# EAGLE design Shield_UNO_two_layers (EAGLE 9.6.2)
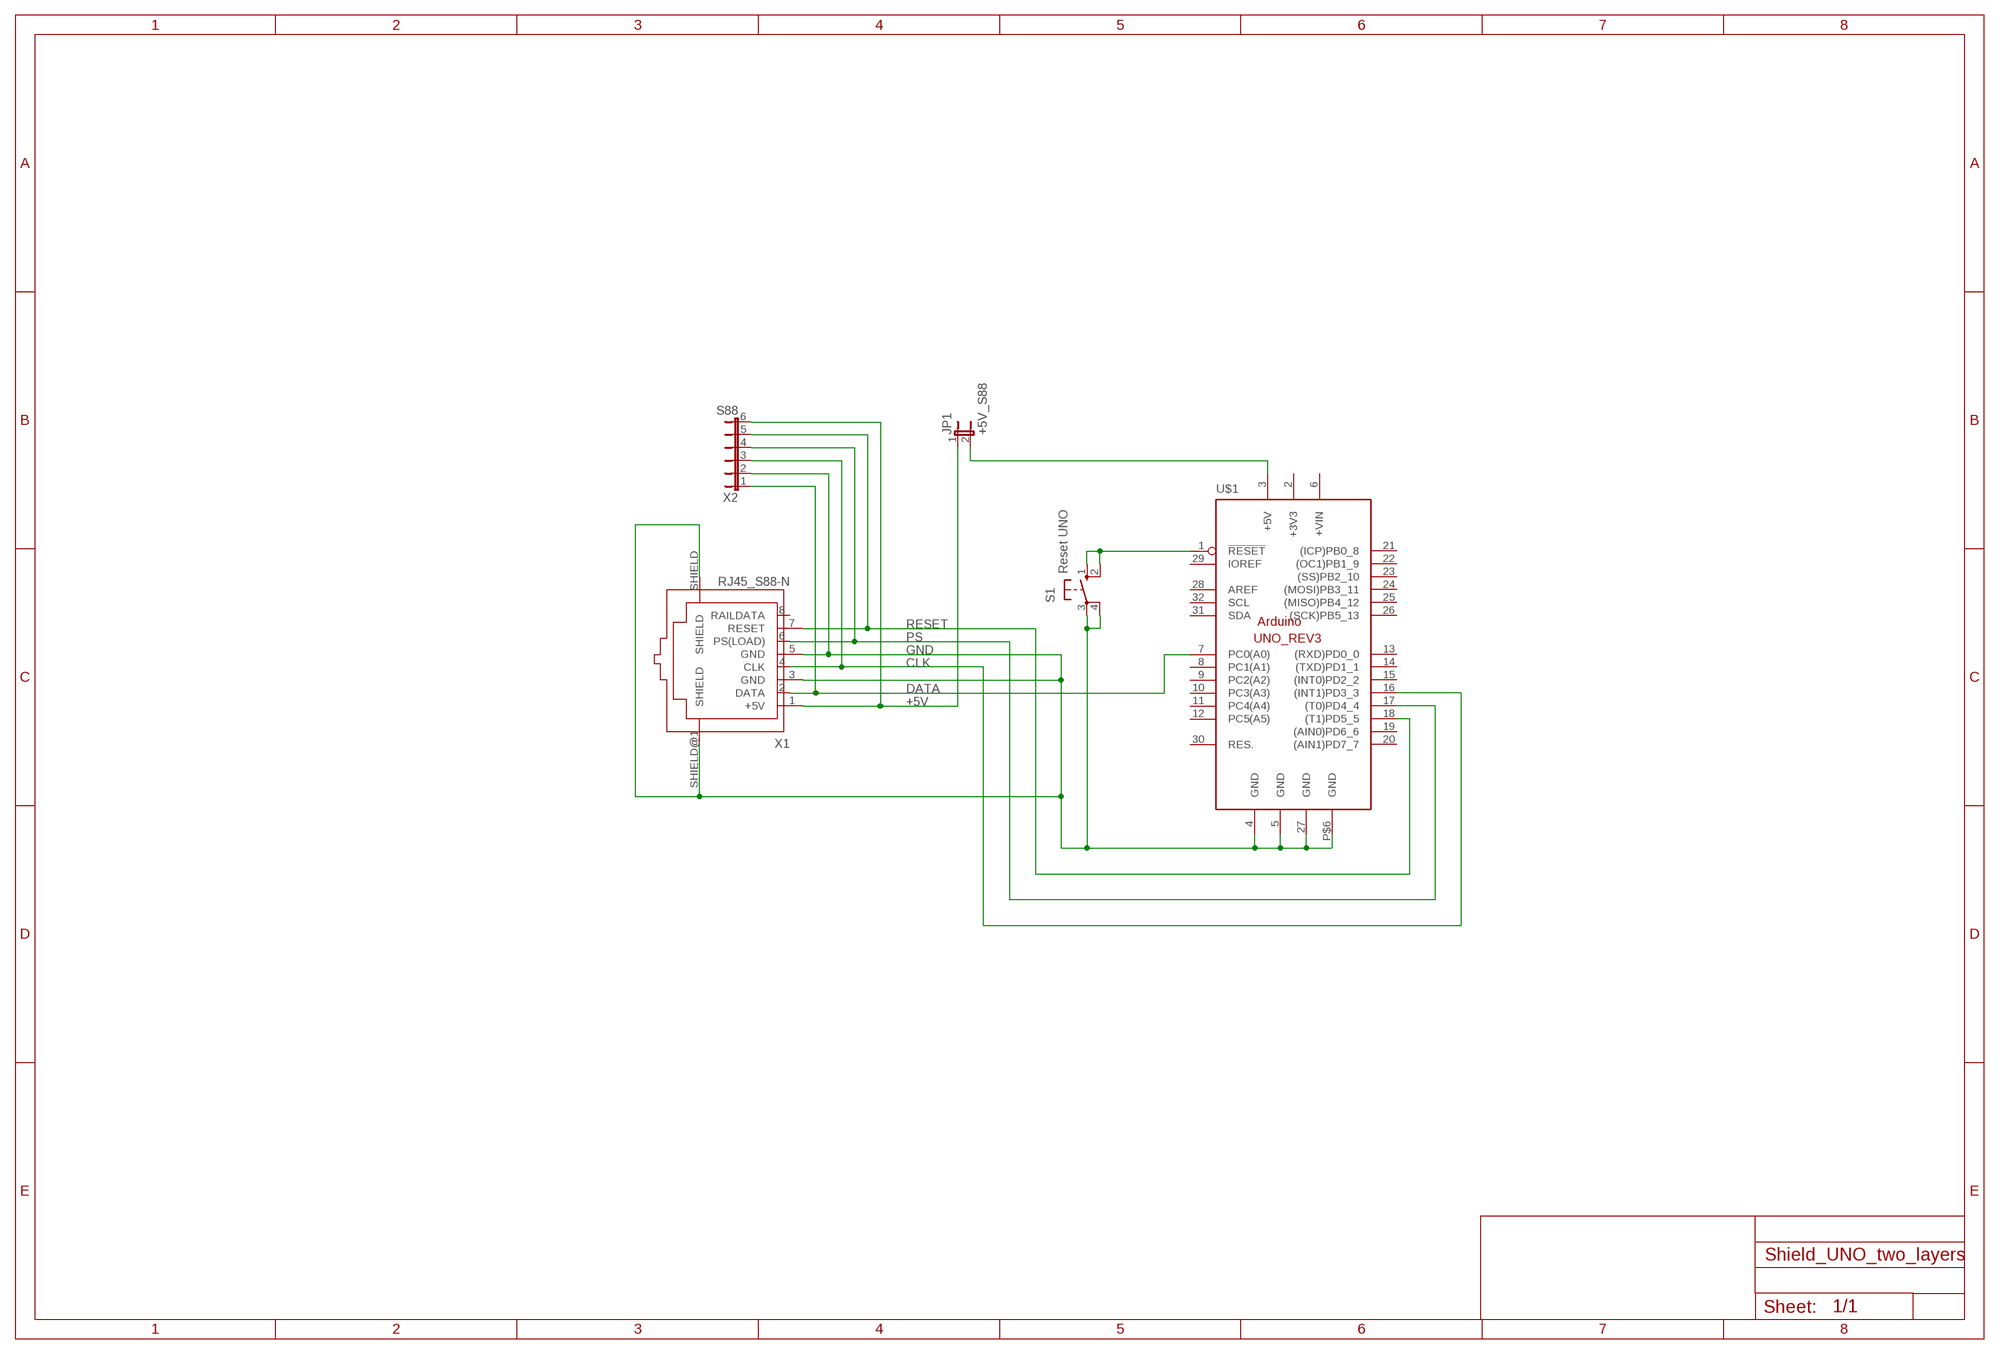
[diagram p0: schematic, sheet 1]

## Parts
JP1  +5V_S88  JP1E  [JP1]
S1  Reset UNO  10-XX  [B3F-10XX]
U$1  ARDUINO_UNO_REV3  [ARDUINO_UNO_REV3_SHORT]
X1  RJ45_S88-N  RJ45-S88-N  [RJ45-SHIELDED]
X2  S88  JP6E  [JP6]

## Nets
+5V: JP1.1 X1.1(+5V) X2.6
CLK: U$1.16((INT1)PD3_3) X1.4(CLK) X2.3
DATA: U$1.7(PC0(A0)) X1.2(DATA) X2.1
GND: S1.3(P) S1.4(P1) U$1.4(GND) U$1.5(GND) U$1.27(GND) U$1.P$6(GND) X1.3(GND) X1.5(GND) X1.SHIELD X1.SHIELD@1(SHIELD) X2.2
N$1: S1.1(S) S1.2(S1) U$1.1(!RESET)
N$3: JP1.2 U$1.3(+5V)
PS: U$1.17((T0)PD4_4) X1.6(PS(LOAD)) X2.4
RESET: U$1.18((T1)PD5_5) X1.7(RESET) X2.5
Unconnected: U$1.6(+VIN) U$1.8(PC1(A1)) U$1.9(PC2(A2)) U$1.10(PC3(A3)) U$1.11(PC4(A4)) U$1.12(PC5(A5)) U$1.13((RXD)PD0_0) U$1.14((TXD)PD1_1) U$1.15((INT0)PD2_2) U$1.19((AIN0)PD6_6) U$1.20((AIN1)PD7_7) U$1.21((ICP)PB0_8) U$1.22((OC1)PB1_9) U$1.23((SS)PB2_10) U$1.24((MOSI)PB3_11) U$1.25((MISO)PB4_12) U$1.26((SCK)PB5_13) U$1.28(AREF) U$1.29(IOREF) U$1.30(RES.) U$1.31(SDA) U$1.32(SCL) X1.8(RAILDATA)

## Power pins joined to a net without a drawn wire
+3V3: U$1.2(+3V3)

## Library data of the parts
JP1 = jumper:JP1E: JUMPER
S1 = switch-omron:10-XX: OMRON SWITCH
U$1 = arduino:ARDUINO_UNO_REV3
X1 = con-amphenol-rj45_S88-N:RJ45-S88-N: RJ45 socket Naming: BEL FUSESS-7188S-A-NF TMESS-7188S-A-NF Datasheet: https://www.belfuse.com/resources/drawings/stewartconnector/dr-stw-ss-7188s-a-nf-ss-7188s-a-nf-50.pdf
X2 = jumper:JP6E: JUMPER

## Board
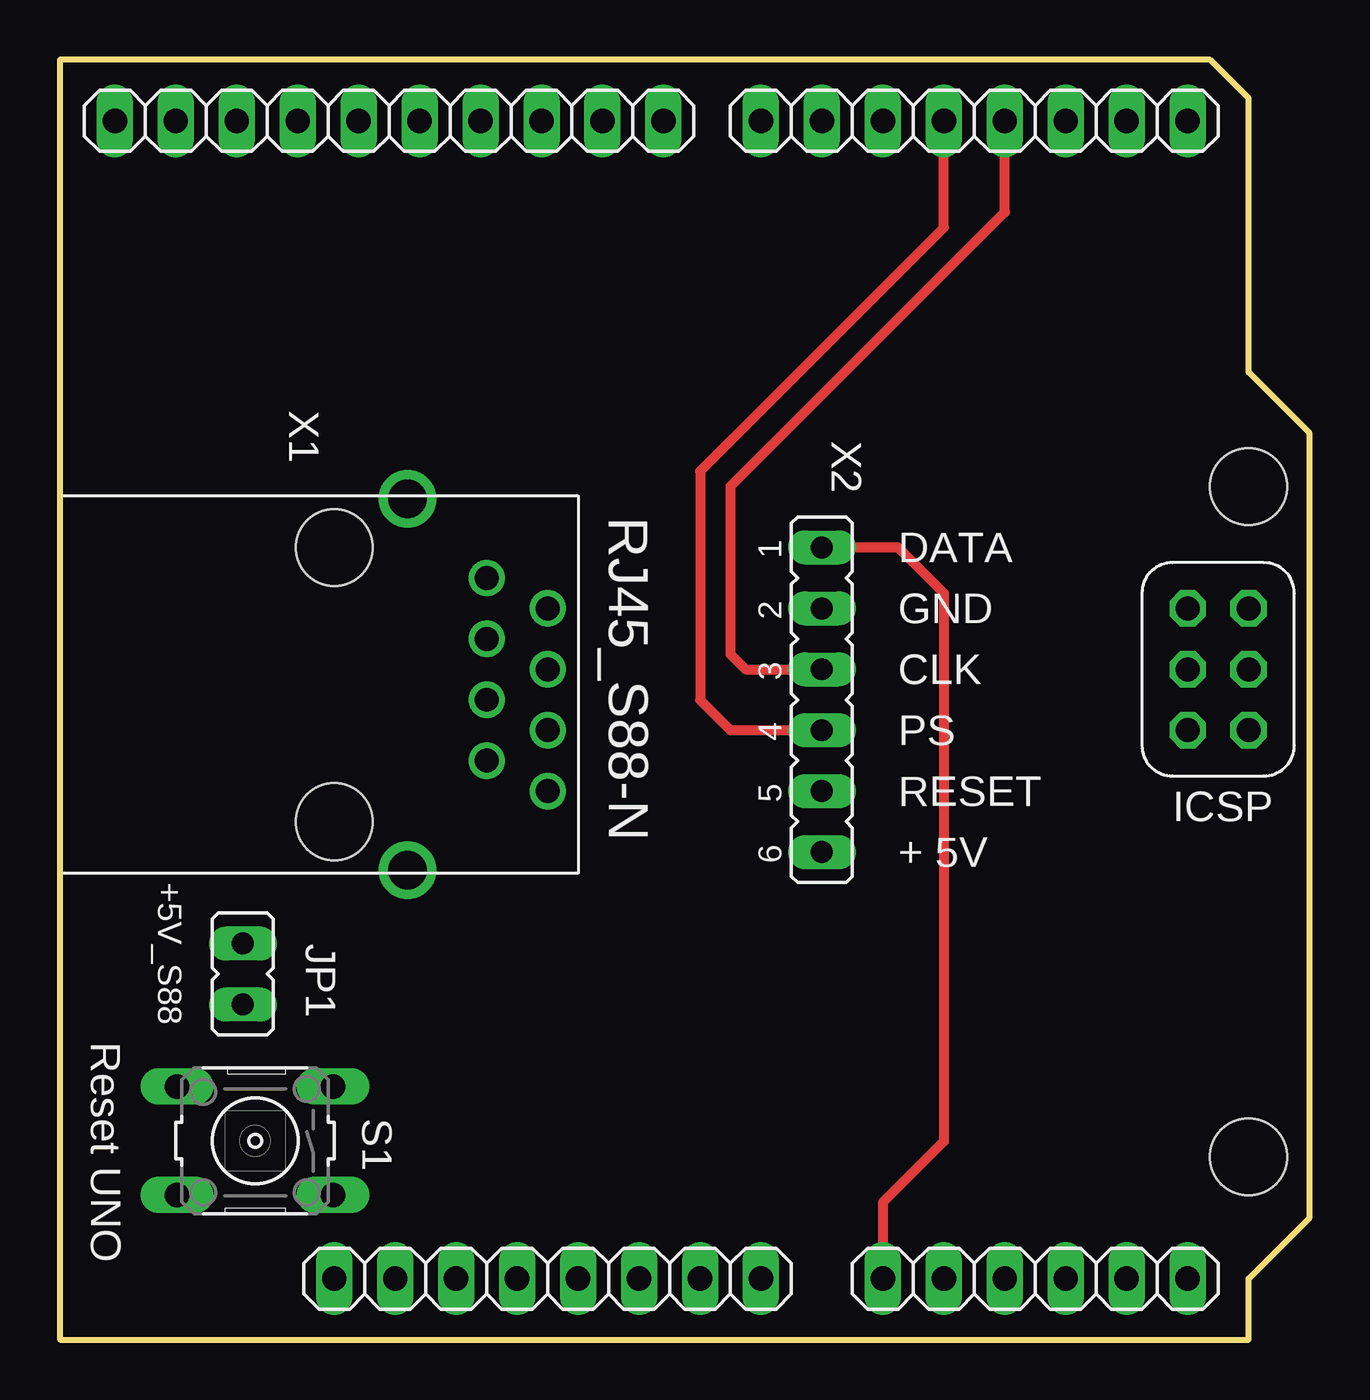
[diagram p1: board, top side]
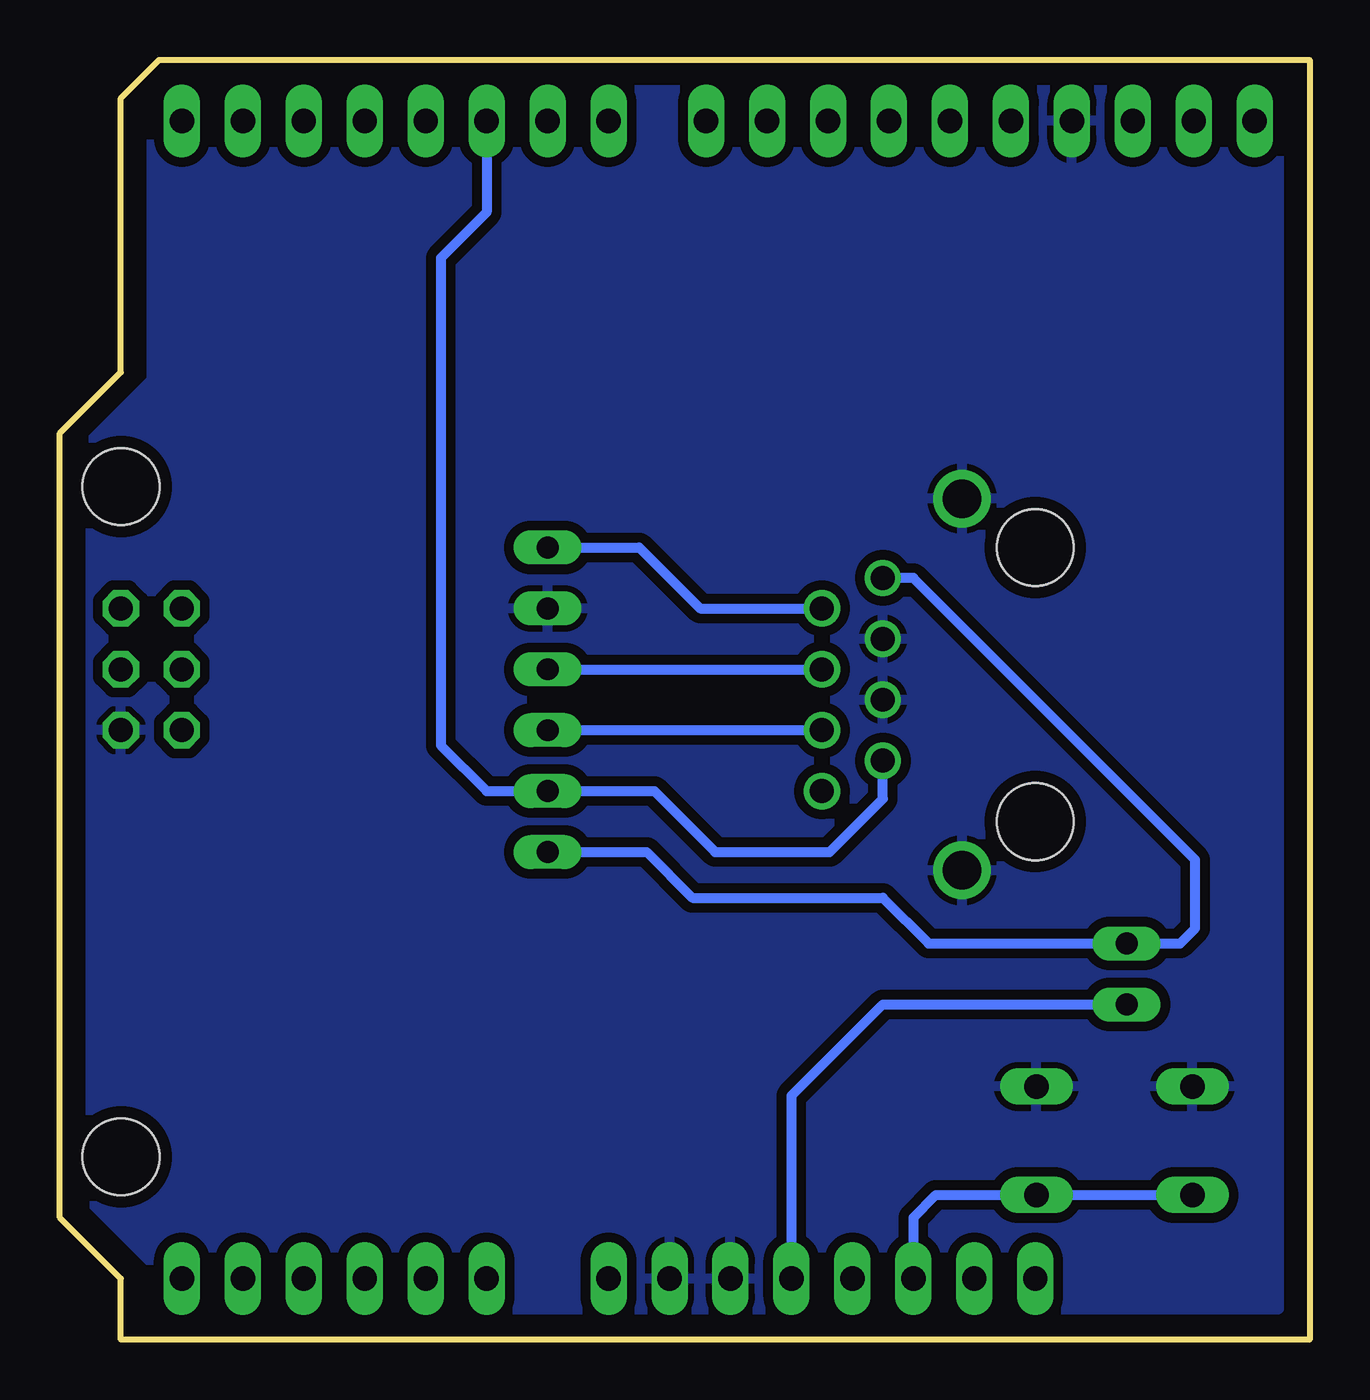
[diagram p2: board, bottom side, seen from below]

Size 52.07 x 53.34 mm. Coordinates in mm from the lower left corner, seen from the top.
Outline: 0,0 49.53,0 49.53,2.54 52.07,5.08 52.07,37.78 49.53,40.32 49.53,51.75 47.94,53.34 0,53.34 0,0
Copper layers (1*16): Top 0.035mm / dielectric 1.5mm / Bottom 0.035mm
Design rules "default *": minimum track width 16mil, minimum drill 20mil, track to track 16mil, track to pad 13mil, pad to pad 16mil, via to via 16mil, smd to smd 10mil, copper to edge 20mil, drill to drill 20mil, minimum pad ring 10mil, minimum via ring 8mil, stop-mask expansion 4mil, vias tented up to drill 0mil, thermal gap 10mil

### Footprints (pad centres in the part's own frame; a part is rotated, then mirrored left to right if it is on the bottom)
JP1 = drill 0.914 long: 1 0,-1.27; 2 0,1.27
B3F-10XX = drill 1.016 long: 1 -3.251,2.261; 2 3.251,2.261; 3 -3.251,-2.261; 4 3.251,-2.261
ARDUINO_UNO_REV3_SHORT = drill 1.016 long: 1 16.51,2.54; 2 19.05,2.54; 3 21.59,2.54; 4 24.13,2.54; 5 26.67,2.54; 6 29.21,2.54; 7 34.29,2.54; 8 36.83,2.54; 9 39.37,2.54; 10 41.91,2.54; 11 44.45,2.54; 12 46.99,2.54; 13 46.99,50.8; 14 44.45,50.8; 15 41.91,50.8; 16 39.37,50.8; 17 36.83,50.8; 18 34.29,50.8; 19 31.75,50.8; 20 29.21,50.8; 21 25.146,50.8; 22 22.606,50.8; 23 20.066,50.8; 24 17.526,50.8; 25 14.986,50.8; 26 12.446,50.8; 27 9.906,50.8; 28 7.366,50.8; 29 13.97,2.54; 30 11.43,2.54; 31 4.826,50.8; 32 2.286,50.8 | drill 1 octagon: P$1 46.99,30.48; P$2 49.53,30.48; P$3 49.53,27.94; P$4 46.99,27.94; P$5 46.99,25.4; P$6 49.53,25.4 | hole 3.2: 49.53,35.56; 49.53,7.62
RJ45-SHIELDED = drill 1: 1 -5.08,7.62; 2 -3.81,10.16; 3 -2.54,7.62; 4 -1.27,10.16; 5 0,7.62; 6 1.27,10.16; 7 2.54,7.62; 8 3.81,10.16 | drill 1.6: SHIELD -8.382,4.318; SHIELD@1 7.112,4.318 | hole 3.2: -6.35,1.27; 5.08,1.27
JP6 = drill 0.914 long: 1 -6.35,0; 2 -3.81,0; 3 -1.27,0; 4 1.27,0; 5 3.81,0; 6 6.35,0

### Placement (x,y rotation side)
JP1  7.62,15.24 180 top
S1  8.13,8.28 180 top
U$1  0,0 0 top
X1  10.16,26.67 270 top
X2  31.75,26.67 270 top

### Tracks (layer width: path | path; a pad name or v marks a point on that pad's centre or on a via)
+5V
  Bottom 0.406: X1.1 16.51,31.75 4.76,20 4.76,17.14 5.4,16.51 JP1.1 15.88,16.51 17.78,18.41 25.72,18.41 27.62,20.32 X2.6
CLK
  Top 0.406: U$1.16 39.37,46.99 27.94,35.56 27.94,28.57 28.57,27.94 X2.3
  Bottom 0.406: X2.3 X1.4
DATA
  Top 0.406: X2.1 34.92,33.02 36.83,31.11 36.83,8.25 34.29,5.72 U$1.7
  Bottom 0.406: X1.2 25.4,30.48 27.94,33.02 X2.1
GND
  pour Bottom: 1.27,52.07 47.62,52.07 48.26,51.43 48.26,40 50.8,37.46 50.8,5.72 48.26,3.17 48.26,1.91 47.62,1.27 1.27,1.27
N$1
  Bottom 0.406: S1.2 S1.1 15.57,6.02 16.51,5.08 U$1.1
N$3
  Bottom 0.406: JP1.2 17.78,13.97 21.59,10.16 U$1.3
PS
  Top 0.406: U$1.17 36.83,46.35 26.67,36.19 26.67,26.67 27.94,25.4 X2.4
  Bottom 0.406: X2.4 X1.6
RESET
  Bottom 0.406: X1.7 17.78,22.54 20,20.32 24.77,20.32 27.3,22.86 X2.5 34.29,22.86 36.2,24.76 36.2,45.08 34.29,46.99 U$1.18

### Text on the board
tNames: DATA | GND | CLK | PS | RESET | + 5V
